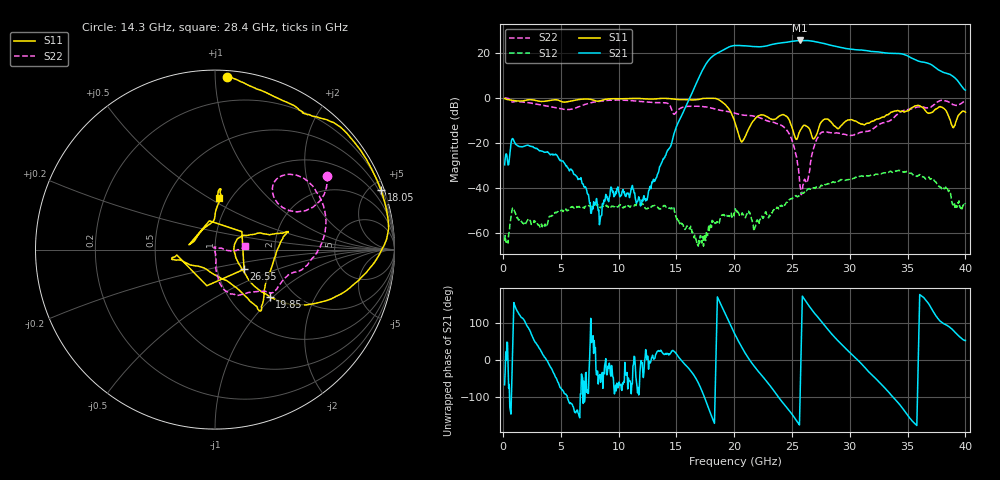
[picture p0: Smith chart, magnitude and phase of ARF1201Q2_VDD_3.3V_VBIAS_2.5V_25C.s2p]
!Bias:VDD=3.3V, VBIAS=2.5V
# GHz S DB R 50.0
!freq dBS11 angS11 dBS21 angS21 dBS12 angS12 dBS22 angS22
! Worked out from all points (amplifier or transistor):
!   798 points, 150 MHz to 40 GHz, reference 50 ohm
!   highest |S21| = 25.6 dB at 25.7 GHz (marker M1)
!   |S21| within 3 dB of that: 19.5 GHz to 29.1 GHz (9.599 GHz wide, 39.5 % of centre)
!   unconditionally stable (mu >= 1): start of sweep to 18.35 GHz; 18.44 GHz to 35.95 GHz; 35.97 GHz to end of sweep
!   at 6.8 GHz: K = 603.04, MAG = -25.0 dB, |S12| = -48.3 dB
!   at 20.1 GHz: K = 7.36, MAG = 24.7 dB, |S12| = -49.3 dB
!   at 40 GHz: K = 14.91, MAG = 10.4 dB, |S12| = -46.8 dB
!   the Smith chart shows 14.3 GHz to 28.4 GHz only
!   S11 on the Smith chart (normalised r, x): 14.3 GHz: 0.04, +1.07; 18.05 GHz: 0.31, +5.76; 19.85 GHz: 1.52, -0.95; 26.55 GHz: 1.35, -0.31; 28.4 GHz: 0.88, +0.55
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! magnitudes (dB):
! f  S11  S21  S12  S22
! 150 MHz  -0.3  -29.8  -63.6  0.0
! 900 MHz  -1.1  -18.4  -49.0  -1.8
! 3.65 GHz  -1.5  -24.2  -56.2  -3.5
! 6.8 GHz  -0.6  -36.7  -48.3  -3.5
! 8.4 GHz  -1.3  -54.6  -48.8  -1.4
! 9.4 GHz  -0.4  -40.0  -48.1  -1.0
! 12.4 GHz  -0.5  -45.1  -49.4  -1.8
! 13.45 GHz  -0.3  -33.2  -49.2  -2.1
! 14.3 GHz  -0.3  -23.2  -48.9  -2.5
! 16.85 GHz  -0.7  7.9  -65.2  -3.7
! 18.05 GHz  -0.2  18.1  -57.6  -4.5
! 19.85 GHz  -7.9  23.2  -52.8  -6.5
! 20.1 GHz  -11.4  23.3  -49.3  -6.8
! 20.7 GHz  -19.4  23.3  -51.2  -7.6
! 22.1 GHz  -8.0  22.8  -55.2  -8.6
! 24.45 GHz  -8.0  24.7  -47.2  -13.7
! 25.7 GHz  -14.6  25.6  -42.7  -39.4
! 26.55 GHz  -14.2  25.4  -40.6  -31.7
! 26.75 GHz  -17.5  25.3  -40.0  -24.7
! 28.4 GHz  -10.8  23.4  -37.9  -15.5
! 33.4 GHz  -7.1  19.9  -32.9  -10.3
! 40 GHz  -6.4  3.5  -46.8  -1.3
